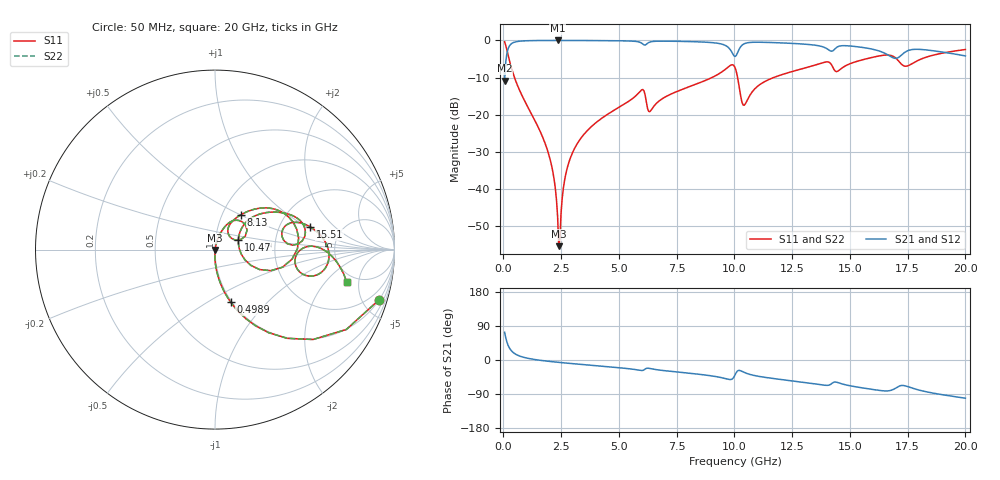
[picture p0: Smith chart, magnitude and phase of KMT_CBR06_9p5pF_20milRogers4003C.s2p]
! Data measured by Modelithics Inc. support@modelithics.com 813-866-6335
! KEMET CBR0603 9.5pF, Pad Width= 0.851mm, Pad Length= 0.64mm, Pad Gap= 0.62mm, 20mil Rogers 4003C substrate Data, January 2022
# hz S ma R 50
! 2 Port Network Data from SP1.SP block
! freq  magS11  angS11  magS21  angS21  magS12  angS12  magS22  angS22
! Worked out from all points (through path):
!   401 points, 50 MHz to 20 GHz, reference 50 ohm
!   highest |S21| = -0.01 dB at 2.344 GHz (marker M1); lowest = -10.8 dB at 50 MHz (marker M2)
!   group delay of S21, straight-line fit = 14.5 ps
!   lowest |S11| = -55.4 dB at 2.394 GHz (marker M3), VSWR 1.00, Z = 50.1 - j0.131 ohm
!   |S11| at or under -10 dB: 479.4 MHz to 9.023 GHz (8.543 GHz wide, 180 % of centre); 10.14 GHz to 11.69 GHz (1.557 GHz wide, 14.3 % of centre)
!   |S22| runs from -55.4 to -0.4 dB; largest |S21 - S12| = 0
!   S11 on the Smith chart (normalised r, x): 50 MHz: 0.99, -6.59; 498.9 MHz: 0.99, -0.63; 8.13 GHz: 1.23, +0.51; 10.47 GHz: 1.29, +0.14; 15.51 GHz: 2.97, +1.07; 20 GHz: 4.18, -3.46
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5e7  0.9575 -16.9  0.2882 73.1  0.2882 73.1  0.9575 -16.9
2.99375e8  0.4794 -62.1  0.8769 27.9  0.8769 27.9  0.4794 -62.1
4.98875e8  0.3039 -73.5  0.9519 16.4  0.9519 16.4  0.3039 -73.5
1.895375e9  0.03411 -91.2  0.9982 -3.0  0.9982 -3.0  0.03411 -91.2
2.194625e9  0.01345 -89.9  0.9986 -5.0  0.9986 -5.0  0.01345 -89.9
2.34425e9  0.004315 -79.4  0.9987 -5.9  0.9987 -5.9  0.004315 -79.4
2.394125e9  0.001706 -49.8  0.9987 -6.2  0.9987 -6.2  0.001706 -49.8
2.793125e9  0.02085 77.8  0.9984 -8.5  0.9984 -8.5  0.02085 77.8
3.391625e9  0.05016 76.5  0.9971 -11.8  0.9971 -11.8  0.05016 76.5
5.93525e9  0.2094 50.9  0.9361 -27.4  0.9361 -27.4  0.2094 50.9
6.33425e9  0.1101 43.2  0.9492 -22.4  0.9492 -22.4  0.1101 43.2
6.73325e9  0.1527 59.4  0.977 -26.4  0.977 -26.4  0.1527 59.4
8.12975e9  0.2438 53.2  0.9634 -35.4  0.9634 -35.4  0.2438 53.2
9.576125e9  0.4017 34.1  0.8652 -48.5  0.8652 -48.5  0.4017 34.1
1.0025e10  0.4326 -7.1  0.6076 -39.7  0.6076 -39.7  0.4326 -7.1
1.047388e10  0.1403 21.9  0.9142 -34.0  0.9142 -34.0  0.1403 21.9
1.127188e10  0.275 40.9  0.9431 -45.3  0.9431 -45.3  0.275 40.9
1.336662e10  0.4537 25.9  0.8721 -61.8  0.8721 -61.8  0.4537 25.9
1.551125e10  0.5451 13.5  0.8076 -73.3  0.8076 -73.3  0.5451 13.5
1.670825e10  0.6336 -6.6  0.6217 -81.0  0.6217 -81.0  0.6336 -6.6
1.74065e10  0.4494 -7.3  0.701 -68.3  0.701 -68.3  0.4494 -7.3
2e10  0.7544 -13.7  0.6184 -100.8  0.6184 -100.8  0.7544 -13.7
